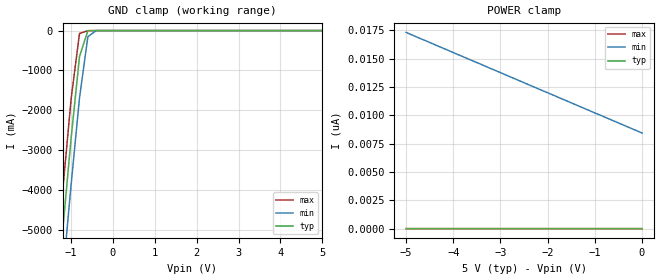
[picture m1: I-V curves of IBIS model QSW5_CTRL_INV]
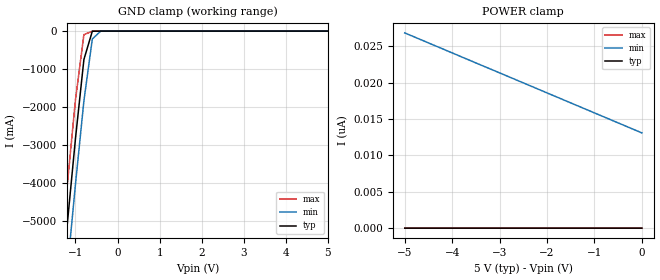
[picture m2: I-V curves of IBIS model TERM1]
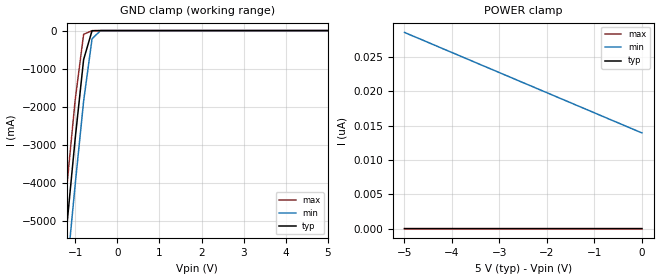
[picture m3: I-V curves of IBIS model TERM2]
| I/O Buffer Information Specification (IBIS) Version 3.2 (August 20, 1999)
| IBIS is a standard for electronic behavioral specifications of integrated
| circuit input/output analog characteristics.
[IBIS Ver]   3.2
[File Name]   qs3l384.ibs
[File Rev]   1.0
[Date]   Wednesday, June 9, 2004
[Source]   Integrated Device Technology, Inc.
[Notes]   1.Temperatures: typ=25C, min=-40C, max=100C
[Disclaimer]
Integrated Device Technology, Inc. ("IDT") hereby grants the user of this
IBIS model ("User") a non-exclusive, nontransferable license to use this
IBIS model under the following terms: The User is granted this license only
to use the IBIS model for demonstration purposes only and is not granted
rights to sell, copy (except as needed to run the IBIS model), rent, lease
or sub-license (except for demonstration) the IBIS model in whole or in
part, or in modified form to anyone. The User may modify the IBIS model to
suit its specific applications, but  rights to derivative works and such
modifications shall belong to IDT.
THIS IBIS MODEL IS PROVIDED ON AN AS IS" BASIS AND IDT  MAKES ABSOLUTELY NO
WARRANTY WITH RESPECT TO THE INFORMATION CONTAINED HEREIN.  IDT DISCLAIMS
AND USER WAIVES ALL WARRANTIES, EXPRESS AND IMPLIED, INCLUDING WARRANTIES OF
MERCHANTABILITY AND FITNESS FOR A PARTICULAR PURPOSE.  THE ENTIRE RISK AS TO
QUALITY AND PERFORMANCE IS WITH THE USER  ACCORDINGLY, IN NO EVENT SHALL IDT
BE LIABLE FOR ANY DIRECT OR INDIRECT DAMAGES, WHETHER IN CONTRACT OR TORT,
INCLUDING ANY LOST PROFITS OR OTHER INCIDENTAL, CONSEQUENTIAL, EXEMPLARY, OR
PUNITIVE DAMAGES ARISING OUT OF THE USE OR APPLICATION OF THE  IBIS MODEL,
WHETHER OR NOT IDT HAD NOTICE OF SUCH DAMAGES.
IDT reserves the right to make changes without notice to any product herein
to improve reliability, function, or design. IDT does not convey any license
under patent rights or any other intellectual property rights, including those
of third parties. IDT is not obligated to provide maintenance or support for
the licensed IBIS model.
This model is for High-Speed Low Power CMOS 10-Bit Bus Switch.
[Copyright]
Copyright 2002, Integrated Device Technology, Inc. All rights reserved.
|   Component qs3l384
[Component]   qs3l384
[Manufacturer]   Integrated Device Technology
[Package]
|Following package parameters are for TSSOP 24 lead package
| variable   typ   min   max
R_pkg   2.500m   2.44m   3.00m
L_pkg   1.00nH   0.91nH   1.74nH
C_pkg   0.17pF   0.16pF   0.27pF
[Pin]  signal_name   model_name   R_pin   L_pin   C_pin
1   _BEA_   QSW5_CTRL_INV
2   B0   TERM2
3   A0   TERM1
4   A1   TERM1
5   B1   TERM2
6   B2   TERM2
7   A2   TERM1
8   A3   TERM1
9   B3   TERM2
10   B4   TERM1
11   A4   TERM1
12   GND   GND
13   _BEB_   QSW5_CTRL_INV
14   A5   TERM1
15   B5   TERM2
16   B6   TERM2
17   A6   TERM1
18   A7   TERM1
19   B7   TERM2
20   B8   TERM2
21   A8   TERM1
22   A9   TERM1
23   B9   TERM2
24   VCC   POWER
[Series Switch Groups]
|Function Group States
On A /
On B /
On A B /
Off A B /
[Series Pin Mapping]   pin_2   model_name   function_table_group
3   2   QSW5_SW   A
4   5   QSW5_SW   A
7   6   QSW5_SW   A
8   9   QSW5_SW   A
11   10   QSW5_SW   A
14   15   QSW5_SW   B
17   16   QSW5_SW   B
18   19   QSW5_SW   B
21   20   QSW5_SW   B
22   23   QSW5_SW   B
|   Model QSW5_SW
[Model]   QSW5_SW
Model_type   Series_switch
C_comp   0.0pF   0.0pF   0.0pf
[Temperature Range]   25.00   100.00   -40.00
[Voltage Range]   5.00V   4.75V   5.25V
[On]
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[Off]
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| Models and submodels in the file (4): QSW5_CTRL_INV (Input), TERM1 (Terminator), TERM2 (Terminator), QSW5_SW (Series_switch)
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|   Model QSW5_CTRL_INV
[Model]   QSW5_CTRL_INV
Model_type   Input
Vinl =  0.80000V
Vinh =  2.00000V
C_comp   4.20000pF   4.20000pF   4.20000pF
[Temperature Range]   25.00000   100.00000   -40.00000
[Voltage Range]   5.00000V   4.75000V   5.25000V
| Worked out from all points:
|   GND clamp passes 1 mA (typ) near -0.48 V on its own axis
[GND_clamp]
| voltage   I(typ)   I(min)   I(max)
-5V       -51.74A    -52.8A     -50.85A
-1.4V     -7.368A    -8.538A    -6.375A
-1.2V     -4.993A    -6.169A    -3.993A
-1V       -2.692A    -3.858A    -1.708A
-800mV    -650.1mA   -1.689A    -70.61mA
-600mV    -2.541mA   -153.7mA   -3.31mA
-400mV    -3.914uA   -449.3uA   -30.03uA
5V        2.373pA    8.883nA    568.4fA
[POWER_clamp]
| voltage   I(typ)   I(min)   I(max)
-5V       3.268pA    17.31nA    739fA
-3.9V     3.055pA    15.35nA    710.5fA
-3.5V     2.998pA    14.65nA    682.1fA
0V        2.373pA    8.439nA    568.4fA
|   Model TERM1
[Model]   TERM1
Model_type   Terminator
Vinl =  0.80000V
Vinh =  2.00000V
C_comp   5.00000pF   5.00000pF   5.00000pF
[Temperature Range]   25.00000   100.00000   -40.00000
[Voltage Range]   5.00000V   4.75000V   5.25000V
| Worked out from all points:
|   GND clamp passes 1 mA (typ) near -0.45 V on its own axis
[GND_clamp]
| voltage   I(typ)   I(min)   I(max)
-5V       -51.88A    -52.98A    -50.96A
-1.4V     -7.503A    -8.707A    -6.481A
-1.2V     -5.126A    -6.335A    -4.097A
-1V       -2.818A    -4.018A    -1.804A
-800mV    -746.5mA   -1.833A    -93.17mA
-600mV    -3.766mA   -208.1mA   -3.113mA
-400mV    -5.035uA   -696.6uA   -28.21uA
5V        2.878pA    13.78nA    632.4fA
[POWER_clamp]
| voltage   I(typ)   I(min)   I(max)
-5V       4.235pA    26.84nA    852.7fA
-3.3V     3.78pA     22.16nA    810fA
-2.3V     3.51pA     19.42nA    753.2fA
0V        2.878pA    13.09nA    639.5fA
|   Model TERM2
[Model]   TERM2
Model_type   Terminator
Vinl =  0.80000V
Vinh =  2.00000V
C_comp   5.70000pF   5.70000pF   5.70000pF
[Temperature Range]   25.00000   100.00000   -40.00000
[Voltage Range]   5.00000V   4.75000V   5.25000V
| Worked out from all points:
|   GND clamp passes 1 mA (typ) near -0.45 V on its own axis
[GND_clamp]
| voltage   I(typ)   I(min)   I(max)
-5V       -51.9A     -53A       -50.97A
-1.4V     -7.523A    -8.731A    -6.496A
-1.2V     -5.145A    -6.358A    -4.111A
-1V       -2.836A    -4.04A     -1.818A
-800mV    -760.6mA   -1.854A    -96.89mA
-600mV    -3.962mA   -216.8mA   -3.113mA
-400mV    -5.095uA   -741.2uA   -28.21uA
5V        2.956pA    14.67nA    632.4fA
[POWER_clamp]
| voltage   I(typ)   I(min)   I(max)
-5V       4.377pA    28.57nA    852.7fA
-4.2V     4.15pA     26.22nA    838.4fA
-3.9V     4.064pA    25.35nA    824.2fA
0V        2.956pA    13.94nA    639.5fA
